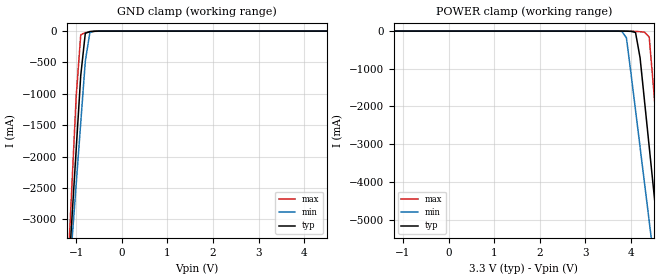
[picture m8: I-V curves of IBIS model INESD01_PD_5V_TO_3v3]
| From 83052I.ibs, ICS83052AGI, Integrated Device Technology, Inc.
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[Model] INESD01_PD_5V_TO_3v3
Model_type   Input
Polarity   Non-Inverting
Vinl = 0.8V
Vinh = 2.0V
|   typ   min   max
C_comp   2pF   1.5pF   2.5pF
|   typ   min   max
[Voltage range]  3.3V   3.135V   3.465V
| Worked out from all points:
|   GND clamp passes 1 mA (typ) near -0.54 V on its own axis
[GND_clamp]
|Voltage I(typ)   I(min)   I(max)
-3.3V     -29.05A    -25.05A    -35.74A
-1.2V     -4.246A    -4.402A    -4.061A
-1.1V     -3.066A    -3.421A    -2.553A
-1V       -1.886A    -2.44A     -1.044A
-900mV    -707.1mA   -1.46A     -57.39mA
-800mV    -35.57mA   -480.7mA   -24.35mA
-700mV    -6.978mA   -23.99mA   -13.24mA
-600mV    -2.058mA   -1.658mA   -4.859mA
6.6V      128.6uA    160.8uA    121.8uA
[POWER_clamp]
|Voltage   I(typ)   I(min)   I(max)
-3.3V     128.6uA    156.8uA    124.8uA
3.8V      -351.6uA   -8.794mA   -15.97uA
3.9V      -2.058mA   -177.5mA   -192.4uA
4.1V      -35.57mA   -2.096A    -7.371mA
4.2V      -707.1mA   -3.077A    -16.88mA
4.3V      -1.886A    -4.058A    -29.22mA
4.4V      -3.066A    -5.04A     -160.2mA
4.5V      -4.246A    -6.022A    -1.572A
4.6V      -5.426A    -7.005A    -3.08A
4.7V      -6.607A    -7.988A    -4.589A
4.8V      -7.788A    -8.97A     -6.098A
6.6V      -29.05A    -26.68A    -33.25A
